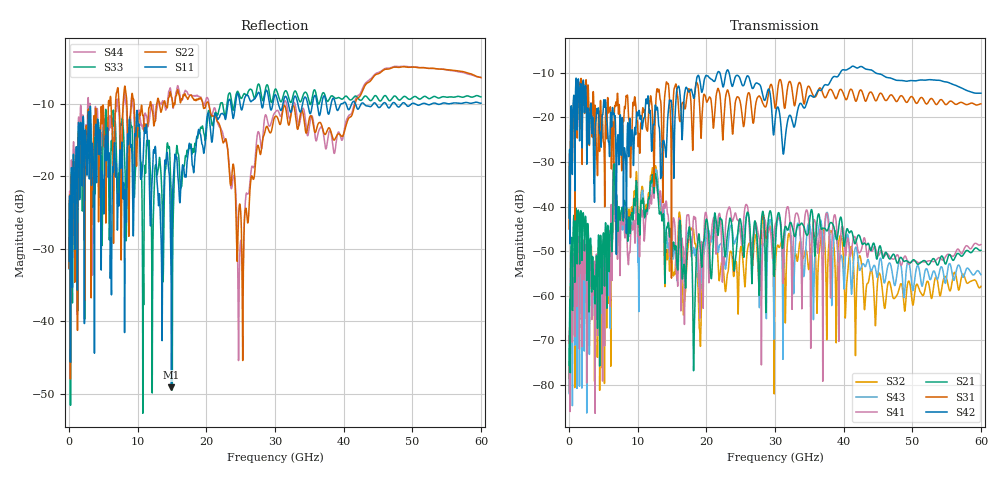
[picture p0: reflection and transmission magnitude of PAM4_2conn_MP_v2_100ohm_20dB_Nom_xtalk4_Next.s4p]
! Info: Touchstone file created by Circ.  Input file=FAB50GbE_2conn_Midplane_Examax_Topo2_v2_100ohm_20dB_Nom.circ
# Hz S RI R 50
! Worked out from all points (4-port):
!   6000 points, 10 MHz to 60 GHz, reference 50 ohm
!   strongest paths, dB at 10 MHz, 15.01 GHz, 30.01 GHz, 45.01 GHz, 60 GHz:
!     S42: -42.6, -18.4, -20.8, -10.2, -14.6
!     S31: -45.0, -24.3, -17.8, -15.5, -16.9
!     S21: -75.6, -51.1, -50.3, -50.6, -49.8
!     S41: -68.0, -47.4, -44.3, -51.0, -48.5
!     S43: -71.0, -49.7, -50.4, -54.9, -55.3
!     S32: -74.8, -53.3, -56.5, -55.9, -57.9
!   lowest |S11| = -49.1 dB at 14.92 GHz (marker M1), VSWR 1.01, Z = 49.9 - j0.333 ohm
!   |S11| at or under -10 dB: start of sweep to 23.14 GHz; 42.96 GHz to 44.31 GHz (1.348 GHz wide, 3.09 % of centre); 44.7 GHz to 45.71 GHz (1.015 GHz wide, 2.25 % of centre)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
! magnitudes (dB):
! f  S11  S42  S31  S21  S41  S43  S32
! 10 MHz  -31.7  -42.6  -45.0  -75.6  -68.0  -71.0  -74.8
! 850 MHz  -29.8  -32.8  -30.0  -55.7  -61.8  -62.2  -65.3
! 6.69 GHz  -16.4  -19.6  -17.5  -37.5  -42.8  -39.6  -36.6
! 14.92 GHz  -49.1  -16.6  -56.0  -48.1  -44.8  -47.3  -50.5
! 24.87 GHz  -9.7  -11.1  -16.1  -42.7  -44.4  -45.2  -51.0
! 28.66 GHz  -8.2  -15.7  -17.6  -63.3  -44.1  -56.0  -47.2
! 60 GHz  -9.9  -14.6  -16.9  -49.8  -48.5  -55.3  -57.9
